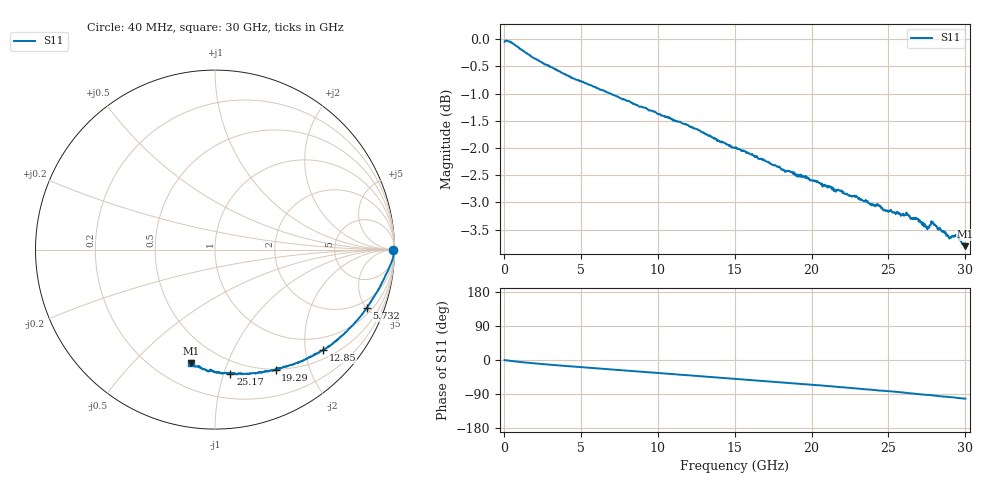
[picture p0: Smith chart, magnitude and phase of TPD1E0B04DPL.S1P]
!  1-Port S-parameters saved by WinCal
! VAR MeasName=S-Parameters (CALIBRATED_DATA) read from VNA (37369D)
! VAR MeasDate=4/29/2016 12:05:45 PM
! VAR NAME=TPD1E0B04DPL
! VAR FILENAME=TPD1E0B04DPL.S1P
! VAR DATE=4/29/2016 12:05:45 PM
! VAR PHYS_PORTS=1
! VAR ObjTypeName=DATASET
! VAR IndexType=Frequency
! Port data:
!!!Port 1: Pin 1_In
# Hz S MA R 50
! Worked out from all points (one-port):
!   801 points, 40 MHz to 30 GHz, reference 50 ohm
!   lowest |S11| = -3.8 dB at 30 GHz (marker M1), VSWR 4.64, Z = 17.3 - j37.5 ohm
!   |S11| at or under -10 dB: nowhere
!   S11 on the Smith chart (normalised r, x): 40 MHz: open; 5.732 GHz: 1.37, -5.00; 12.85 GHz: 0.69, -2.38; 19.29 GHz: 0.49, -1.51; 25.17 GHz: 0.39, -1.05; 30 GHz: 0.35, -0.75
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4e7  0.9945 -0.2
3.396e8  0.995 -1.8
7.5155e8  0.9863 -3.9
1.4631e9  0.9707 -6.9
2.39935e9  0.9531 -10.3
3.82245e9  0.93 -15.2
5.7324e9  0.9061 -21.1
7.56745e9  0.8825 -26.8
9.1029e9  0.8652 -31.5
1.131245e10  0.84 -38.4
1.28479e10  0.8218 -42.9
1.505745e10  0.7953 -49.8
1.68176e10  0.7747 -55.4
1.8765e10  0.7554 -61.4
1.92893e10  0.751 -63.3
2.052515e10  0.7374 -66.9
2.179845e10  0.7262 -71.4
2.254745e10  0.7176 -74.0
2.434505e10  0.7032 -80.5
2.516895e10  0.6966 -82.9
2.629245e10  0.6889 -87.1
2.704145e10  0.6817 -90.4
2.74534e10  0.6732 -91.8
2.794025e10  0.6752 -93.7
2.84271e10  0.6666 -96.1
2.898885e10  0.6564 -97.9
2.94008e10  0.659 -99.8
3e10  0.6453 -102.0
